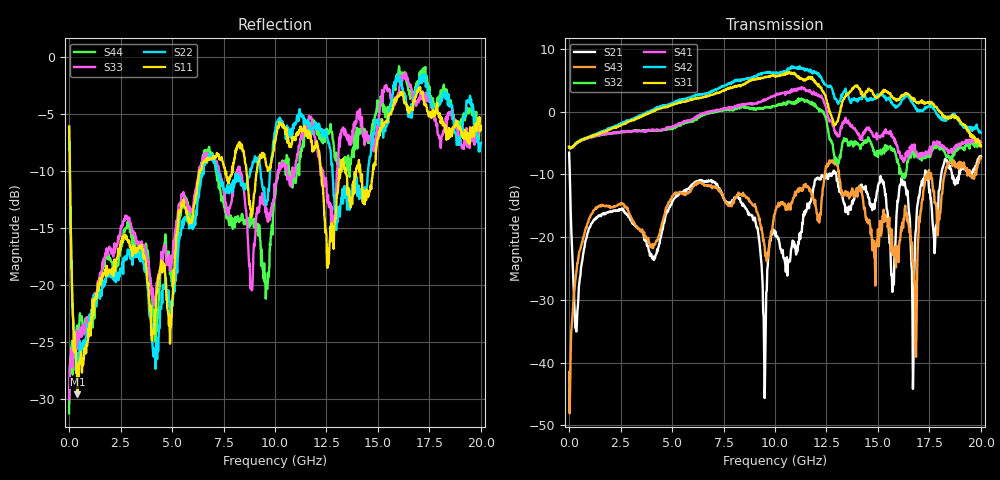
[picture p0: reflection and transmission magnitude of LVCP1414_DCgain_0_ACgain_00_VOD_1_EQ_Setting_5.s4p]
!Agilent Technologies,N5230A,MY46400459,A.07.50.48
!Agilent N5230A: A.07.50.48
!Date: Tuesday, April 17, 2012 18:27:24
!Correction: S11(Full 4 Port(1,2,3,4))
!S12(Full 4 Port(1,2,3,4))
!S13(Full 4 Port(1,2,3,4))
!S14(Full 4 Port(1,2,3,4))
!S21(Full 4 Port(1,2,3,4))
!S22(Full 4 Port(1,2,3,4))
!S23(Full 4 Port(1,2,3,4))
!S24(Full 4 Port(1,2,3,4))
!S31(Full 4 Port(1,2,3,4))
!S32(Full 4 Port(1,2,3,4))
!S33(Full 4 Port(1,2,3,4))
!S34(Full 4 Port(1,2,3,4))
!S41(Full 4 Port(1,2,3,4))
!S42(Full 4 Port(1,2,3,4))
!S43(Full 4 Port(1,2,3,4))
!S44(Full 4 Port(1,2,3,4))
!S4P File: Measurements: <S11,S12,S13,S14>,
!<S21,S22,S23,S24>,
!<S31,S32,S33,S34>,
!<S41,S42,S43,S44>:
# Hz S  dB  R 50
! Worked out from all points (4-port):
!   801 points, 300 kHz to 20 GHz, reference 50 ohm
!   strongest paths, dB at 300 kHz, 5 GHz, 10 GHz, 15 GHz, 20 GHz:
!     S31: -5.6, 1.1, 5.6, 2.3, -5.5
!     S42: -5.7, 1.4, 6.1, 2.5, -3.4
!     S41: -5.6, -2.4, 2.4, -3.8, -4.9
!     S32: -5.7, -2.7, 0.8, -7.2, -5.5
!     S43: -41.5, -13.5, -16.2, -18.7, -7.5
!     S21: -6.5, -14.4, -19.7, -11.9, -7.1
!   lowest |S11| = -29.5 dB at 400.3 MHz (marker M1), VSWR 1.07, Z = 53.1 + j1.41 ohm
!   |S11| at or under -10 dB: 37.63 MHz to 6.365 GHz (6.328 GHz wide, 198 % of centre); 12.22 GHz to 13.12 GHz (896.1 MHz wide, 7.07 % of centre); 14.14 GHz to 14.76 GHz (611.9 MHz wide, 4.23 % of centre)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
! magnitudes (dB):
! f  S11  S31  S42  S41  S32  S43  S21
! 300 kHz  -6.1  -5.6  -5.7  -5.6  -5.7  -41.5  -6.5
! 400.3 MHz  -29.5  -4.9  -4.9  -5.0  -4.9  -24.1  -31.8
! 10 GHz  -7.5  5.6  6.1  2.4  0.8  -16.2  -19.7
! 12.88 GHz  -15.0  -2.2  2.5  -3.0  -6.8  -8.0  -9.7
! 16.8 GHz  -3.6  1.8  0.9  -5.9  -6.7  -28.9  -20.9
! 17.4 GHz  -4.8  1.5  0.8  -6.8  -6.5  -10.1  -9.7
! 20 GHz  -6.4  -5.5  -3.4  -4.9  -5.5  -7.5  -7.1
